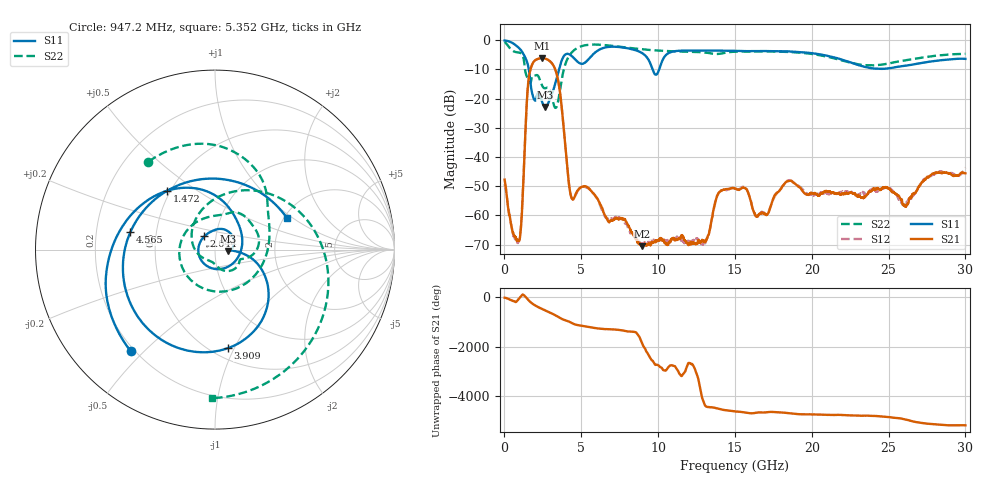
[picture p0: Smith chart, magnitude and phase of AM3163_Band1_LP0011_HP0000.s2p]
!Agilent Technologies,E8364B,MY43040894,A.07.50.67
!Agilent E8364B: A.07.50.67
!Date: Thursday, August 20, 2020 11:23:15
!Correction: S11(Full 2 Port(1,2))
!S21(Full 2 Port(1,2))
!S12(Full 2 Port(1,2))
!S22(Full 2 Port(1,2))
!S2P File: Measurements: S11, S21, S12, S22:
# Hz S  dB  R 50
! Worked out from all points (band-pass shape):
!   3201 points, 10 MHz to 30 GHz, reference 50 ohm
!   highest |S21| = -6.08 dB at 2.447 GHz (marker M1); lowest = -70.6 dB at 8.951 GHz (marker M2)
!   |S21| within 3 dB of the highest: 1.746 GHz to 3.231 GHz (1.484 GHz wide, 59.6 % of centre)
!   lowest |S11| = -22.9 dB at 2.662 GHz (marker M3), VSWR 1.15, Z = 57.7 - j0.962 ohm
!   |S11| at or under -10 dB: 1.586 GHz to 3.552 GHz (1.966 GHz wide, 76.5 % of centre); 9.641 GHz to 10.07 GHz (430.4 MHz wide, 4.37 % of centre)
!   |S22| runs from -23.2 to -0.6 dB; largest |S21 - S12| = 0.0044
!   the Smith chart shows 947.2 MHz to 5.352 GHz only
!   S11 on the Smith chart (normalised r, x): 947.2 MHz: 0.19, -0.46; 1.472 GHz: 0.48, +0.38; 2.044 GHz: 0.88, +0.13; 3.909 GHz: 0.60, -0.95; 4.565 GHz: 0.35, +0.09; 5.352 GHz: 2.07, +0.90
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1e7  -0.07 -8.8  -47.75 -27.8  -49.28 -9.7  -0.56 -26.7
4.879656e8  -0.84 -64.9  -64.81 -138.3  -64.58 178.9  -3.43 -148.7
9.471875e8  -2.67 -129.7  -68.79 -68.3  -68.81 61.8  -4.23 127.1
1.472012e9  -7.48 129.2  -19.71 -58.9  -19.70 -58.8  -12.67 -91.5
2.043697e9  -20.46 128.9  -6.71 1.9  -6.70 1.9  -11.99 27.6
2.446688e9  -21.09 -1.6  -6.08 -122.9  -6.08 -122.9  -15.46 -17.4
2.662241e9  -22.90 -6.7  -6.29 176.3  -6.29 176.2  -16.46 -24.0
3.196438e9  -16.79 -7.0  -8.74 21.0  -8.76 21.0  -21.92 -91.1
3.9087e9  -5.14 -82.4  -33.13 152.4  -33.14 153.0  -9.12 69.1
4.564731e9  -6.35 168.4  -53.76 -21.8  -53.82 -20.7  -3.28 -24.9
5.014581e9  -8.07 86.0  -50.31 -80.1  -50.30 -82.4  -2.04 -65.9
5.351969e9  -7.17 23.7  -50.23 -117.4  -50.47 -118.2  -1.63 -91.3
6.448478e9  -2.62 -104.1  -59.00 147.9  -59.42 147.5  -1.62 -156.0
7.526244e9  -2.35 -175.7  -60.99 106.0  -60.87 101.4  -2.23 154.8
8.950769e9  -4.36 108.5  -70.56 -58.4  -70.17 165.2  -3.09 98.4
1.000979e10  -10.84 109.3  -68.65 126.1  -68.62 -41.8  -3.54 59.2
1.239025e10  -3.52 7.7  -69.50 -16.4  -68.05 -32.3  -3.98 -22.2
1.5005e10  -3.64 -72.2  -50.81 66.3  -50.93 69.4  -3.92 -90.4
2.000958e10  -4.43 163.4  -52.34 -54.4  -53.19 -58.6  -4.70 136.6
2.275554e10  -8.03 60.1  -52.37 -100.1  -52.60 -96.5  -7.98 21.3
2.500479e10  -9.63 -61.9  -50.71 -162.0  -50.77 -164.4  -7.97 -92.1
3e10  -6.38 104.6  -45.60 -136.6  -43.61 -133.4  -4.64 102.4
